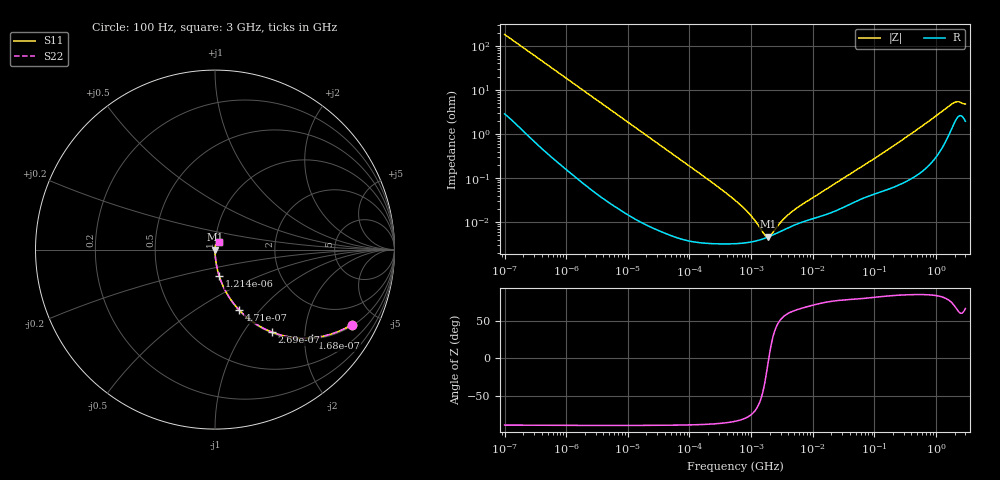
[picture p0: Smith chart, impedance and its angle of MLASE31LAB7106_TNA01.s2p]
! MLASE31LAB7106_TNA01  S-PARAMETER MODEL  ( Standard Model )
! Model Generated by TAIYO YUDEN Corporation (http://www.ty-top.com)
! Version 1.0
! TAIYO YUDEN Control No. 220601
! Copyright(c) 2009 TAIYO YUDEN CO.,LTD. All Rights Reserved.
! Product Description (link to TY-COMPAS)
! https://ds.yuden.co.jp/TYCOMPAS/or/detail?pn=MLASE31LAB7106KTNA01&u=M
! Products Name : Multilayer Ceramic Capacitors
! Characteristics :
!  Capacitance : 10 [uF] , Rated Voltage : 16 [V] , TCC : X7R
!  Case Size : 3.2 x 1.6 / 0.126 x 0.063 [mm/inch] , Thickness : 1.6 / 0.063 [mm/inch]
!  (Conditions: Temperature = 25 [degC] , DC Bias Voltage = 0 [V])
! External Node Assignments :
!  1  o---| |---o  2
! GND o---------o GND
! Frequency Range : 100Hz  -  3GHz  [ 401 STEP ]
# MHZ S RI R 50
! Freq[MHz].  S11 Real  S11 Imag  S21 Real  S21 Imag  S12 Real  S12 Imag  S22 Real  S22 Imag
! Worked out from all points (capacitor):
!   401 points, 100 Hz to 3 GHz, reference 50 ohm
!   read as one part in series: C = 8.76 uF near 109 Hz
!   lowest |Z| = 4.65 mohm at 1.908 MHz (marker M1)
!   series resonance near 1.938 MHz, so ESL is about 770 pH
!   S11 on the Smith chart (normalised r, x): 100 Hz: 1.06, -3.62; 168 Hz: 1.03, -2.17; 269 Hz: 1.02, -1.36; 471 Hz: 1.01, -0.78; 1.214 kHz: 1.00, -0.30; 3 GHz: 1.04, +0.09
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0.0001  0.7627 -0.4176  0.2373 0.4176  0.2373 0.4176  0.7627 -0.4176
0.000168  0.5407 -0.4915  0.4593 0.4915  0.4593 0.4915  0.5407 -0.4915
0.000269  0.3176 -0.4598  0.6824 0.4598  0.6824 0.4598  0.3176 -0.4598
0.000471  0.1341 -0.3359  0.8659 0.3359  0.8659 0.3359  0.1341 -0.3359
0.000724  0.0624 -0.2374  0.9376 0.2374  0.9376 0.2374  0.0624 -0.2374
0.001214  0.0237 -0.148  0.9763 0.148  0.9763 0.148  0.0237 -0.148
0.001788  0.0113 -0.102  0.9887 0.102  0.9887 0.102  0.0113 -0.102
0.005476  0.0014 -0.0338  0.9986 0.0338  0.9986 0.0338  0.0014 -0.0338
0.031977  9.79e-05 -0.00584  0.9999 0.00584  0.9999 0.00584  9.79e-05 -0.00584
0.231582  3.32e-05 -0.000798  1 0.000798  1 0.000798  3.32e-05 -0.000798
0.547723  3.25e-05 -0.000314  1 0.000314  1 0.000314  3.25e-05 -0.000314
0.806856  3.39e-05 -0.00019  1 0.00019  1 0.00019  3.39e-05 -0.00019
1.188587  3.74e-05 -9.59e-05  1 9.59e-05  1 9.59e-05  3.74e-05 -9.59e-05
1.295438  3.86e-05 -7.77e-05  1 7.77e-05  1 7.77e-05  3.86e-05 -7.77e-05
1.908323  4.64e-05 -2.75e-06  1 2.75e-06  1 2.75e-06  4.64e-05 -2.75e-06
3.063887  6.26e-05 8.06e-05  0.9999 -8.06e-05  0.9999 -8.06e-05  6.26e-05 8.06e-05
4.91919  8.46e-05 0.000166  0.9999 -0.000166  0.9999 -0.000166  8.46e-05 0.000166
9.794414  0.000119 0.000331  0.9999 -0.000331  0.9999 -0.000331  0.000119 0.000331
175.1444  0.000589 0.0046  0.9994 -0.0046  0.9994 -0.0046  0.000589 0.0046
1868.531  0.0167 0.0455  0.9833 -0.0455  0.9833 -0.0455  0.0167 0.0455
2219.584  0.0251 0.0463  0.9749 -0.0463  0.9749 -0.0463  0.0251 0.0463
3000  0.0208 0.042  0.9792 -0.042  0.9792 -0.042  0.0208 0.042
